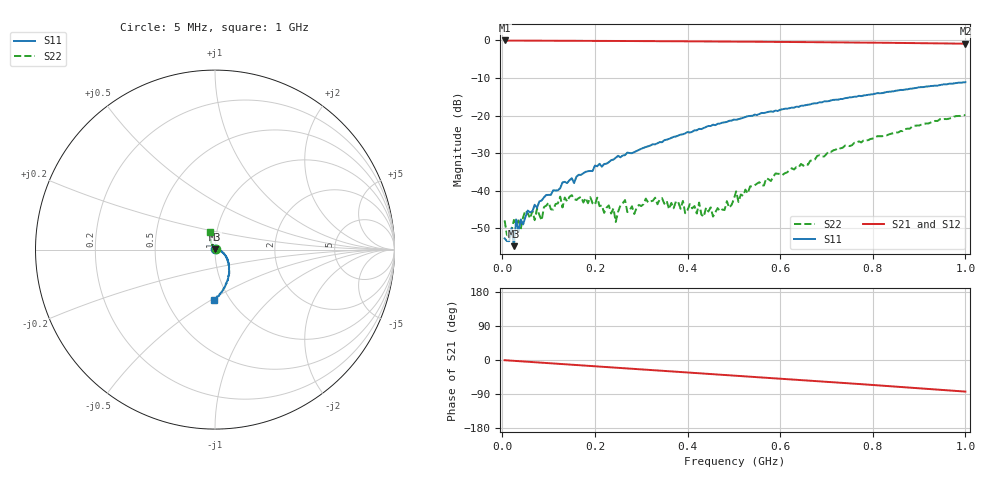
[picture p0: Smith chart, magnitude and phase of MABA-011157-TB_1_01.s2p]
!Agilent Technologies,E5071C,MY46110647,A.11.31
!Date: Fri May 19 08:52:15 2023 DD
!Data & Calibration Information:
!MABA-011157 soldered onto PT-003991 with F connectors, Calibration PCB PT-0003653. Por1 (pin4) Port2 (pin3)
!Freq	S11:SOLT2(ON)	S21:SOLT2(ON)	S12:SOLT2(ON)	S22:SOLT2(ON)
!PortZ  Port1:75+j0  Port2:75+j0
!Above PortZ is port z conversion or system Z0 setting when saving the data.
!When reading, reference impedance value at option line is always used.
# Hz S MA R 75
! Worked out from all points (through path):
!   200 points, 5 MHz to 1 GHz, reference 75 ohm
!   highest |S21| = 0.01 dB at 5 MHz (marker M1); lowest = -0.9 dB at 1 GHz (marker M2)
!   group delay of S21, straight-line fit = 230 ps
!   lowest |S11| = -54.8 dB at 25 MHz (marker M3), VSWR 1.00, Z = 75.2 + j0.165 ohm
!   |S11| at or under -10 dB: start of sweep to end of sweep
!   |S22| runs from -52.3 to -19.8 dB; largest |S21 - S12| = 0.0046
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5000000  0.002318 164.8  1.001 -0.5  0.9981 -0.3  0.004018 22.8
1.5e7  0.002127 38.8  0.9978 -1.3  0.9979 -1.3  0.002438 29.5
2e7  0.003185 10.2  0.9975 -1.7  0.9973 -1.7  0.002986 46.8
2.5e7  0.001824 37.0  0.9969 -2.2  0.997 -2.2  0.004069 30.4
3e7  0.004151 25.0  0.9968 -2.6  0.9965 -2.6  0.00359 41.4
3.5e7  0.002827 28.0  0.9964 -3.0  0.996 -3.0  0.004024 26.9
5.5e7  0.005436 28.3  0.9956 -4.6  0.9952 -4.6  0.004998 20.9
1.25e8  0.01078 16.7  0.9919 -10.3  0.9916 -10.3  0.008334 15.5
1.75e8  0.0171 4.2  0.9896 -14.4  0.9896 -14.4  0.006957 31.2
2.05e8  0.02114 -2.0  0.9879 -16.8  0.9885 -16.8  0.008077 28.9
2.2e8  0.02268 -8.5  0.987 -18.0  0.987 -18.0  0.005057 33.5
2.4e8  0.02597 -8.4  0.9857 -19.7  0.9858 -19.7  0.005805 18.5
2.45e8  0.02744 -9.4  0.9856 -20.1  0.9861 -20.1  0.003828 28.4
2.65e8  0.02973 -10.2  0.9838 -21.7  0.9844 -21.7  0.007517 22.7
2.85e8  0.03267 -13.8  0.9828 -23.3  0.9832 -23.4  0.004891 6.5
3.4e8  0.04437 -19.2  0.979 -27.7  0.9793 -27.8  0.007681 15.2
4.55e8  0.07563 -32.7  0.9702 -37.1  0.9701 -37.1  0.004518 67.1
5.05e8  0.08776 -39.8  0.9659 -41.2  0.9656 -41.2  0.009818 96.5
5.1e8  0.08956 -38.9  0.965 -41.6  0.965 -41.6  0.007089 101.7
6.7e8  0.1447 -56.5  0.9502 -54.9  0.9498 -54.9  0.02528 119.3
8.35e8  0.2079 -73.5  0.9311 -68.9  0.93 -69.0  0.05625 116.0
1e9  0.2786 -90.9  0.9065 -83.4  0.9051 -83.4  0.101 106.2
